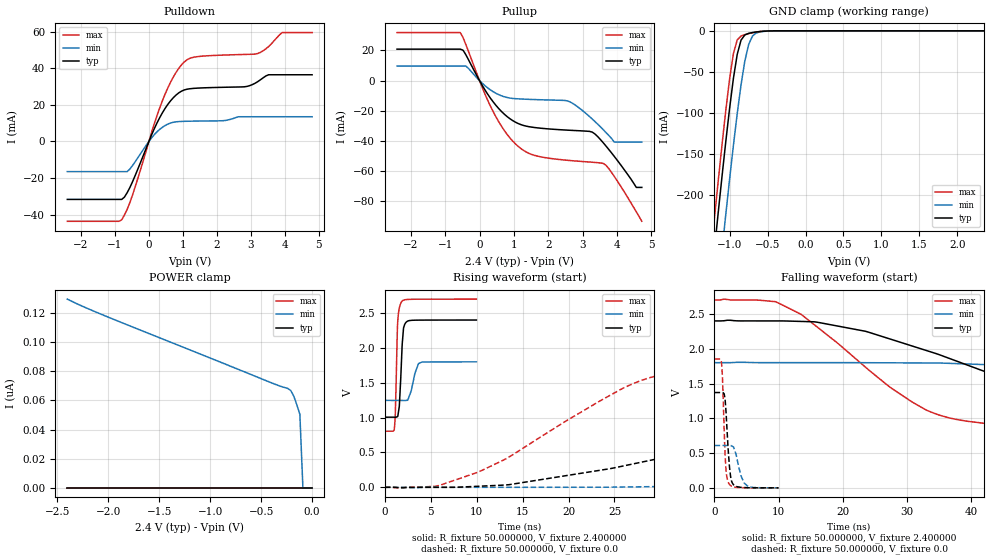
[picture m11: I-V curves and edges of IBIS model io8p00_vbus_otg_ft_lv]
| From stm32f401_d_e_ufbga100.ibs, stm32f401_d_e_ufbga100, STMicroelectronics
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|   Model io8p00_vbus_otg_ft_lv
[Model]  io8p00_vbus_otg_ft_lv
Model_type I/O
Polarity   Non-Inverting
Enable   Active-Low
Vinl =   0.720000V
Vinh =   1.680000V
Vmeas =  1.200000V
Cref =   50.000000pF
Rref =   100.000000M
Vref =   0.0V
C_comp   3.193600pF   3.100000pF   3.332000pF
[Temperature Range]   25.000000   0.125000k   -40.000000
[Pullup Reference]   2.400000V   1.800000V   2.700000V
[Pulldown Reference]   0.0V   0.0V   0.0V
[POWER Clamp Reference]   2.400000V   1.800000V   2.700000V
[GND Clamp Reference]   0.0V   0.0V   0.0V
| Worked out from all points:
|   slope of the pulldown table from 0 to 0.36 V, typ, clamps not added: 25 ohm
|   slope of the pullup table from 0 to 0.36 V, typ, clamps not added: 27.7 ohm
|   GND clamp passes 1 mA (typ) near -0.61 V on its own axis
|   rising waveform, R_fixture 50.000000, V_fixture 2.400000: 20-80 % time 309ps typ, 630ps min, 213ps max; typ from 1.01 V to 2.4 V
|   rising waveform, R_fixture 50.000000, V_fixture 0.0: 20-80 % time 30.9ns typ, 73.2ns min, 14.3ns max; typ from 0 V to 1.37 V
|   falling waveform, R_fixture 50.000000, V_fixture 2.400000: 20-80 % time 29.1ns typ, 72.3ns min, 15.9ns max; typ from 2.4 V to 1.01 V
|   falling waveform, R_fixture 50.000000, V_fixture 0.0: 20-80 % time 575ps typ, 1.04ns min, 436ps max; typ from 1.37 V to 0 V
[Pulldown]
|Voltage   I(typ)   I(min)   I(max)
-2.4V     -31.69mA   -16.5mA    -43.66mA
-800mV    -31.69mA   -16.5mA    -42.82mA
-480mV    -21.96mA   -13.17mA   -29.19mA
80mV      3.63mA     1.966mA    5.014mA
480mV     18.16mA    8.738mA    26.02mA
800mV     25.38mA    10.72mA    37.77mA
1.12V     28.53mA    11.02mA    44.6mA
2.8V      29.84mA    13.49mA    47.53mA
3.2V      32.65mA    13.49mA    48.05mA
3.52V     36.43mA    13.49mA    51.84mA
3.92V     36.43mA    13.49mA    59.49mA
4.8V      36.43mA    13.49mA    59.49mA
[Pullup]
|Voltage   I(typ)   I(min)   I(max)
-2.4V     20.89mA    9.66mA     31.9mA
-560mV    20.89mA    9.66mA     31.9mA
-400mV    17.28mA    9.66mA     24.07mA
320mV     -11.75mA   -6.207mA   -17.08mA
960mV     -26.47mA   -11.82mA   -40.02mA
1.52V     -30.88mA   -12.51mA   -49.05mA
2.56V     -32.88mA   -13.49mA   -52.9mA
3.28V     -34.19mA   -25.52mA   -54.18mA
3.6V      -41.31mA   -32.62mA   -54.99mA
3.92V     -50.33mA   -40.8mA    -63.62mA
4.56V     -70.9mA    -40.8mA    -87.07mA
4.72V     -70.9mA    -40.8mA    -93.4mA
[GND_clamp]
|Voltage   I(typ)   I(min)   I(max)
-2.4V     -1.425A    -1.509A    -1.394A
-1.25V    -311.3mA   -401.9mA   -273.4mA
-1.2V     -265.5mA   -356.1mA   -227.3mA
-1.15V    -220.5mA   -310.9mA   -182mA
-1.1V     -176.4mA   -266.2mA   -138mA
-1.05V    -133.9mA   -222.5mA   -96.06mA
-950mV    -57.51mA   -139mA     -27.35mA
-900mV    -28.55mA   -100.5mA   -11.03mA
-850mV    -11.33mA   -65.67mA   -6.322mA
-750mV    -3.069mA   -16.69mA   -3.425mA
-600mV    -864.6uA   -1.294mA   -852.2uA
2.35V     0A         0A         0A
[POWER_clamp]
|Voltage   I(typ)   I(min)   I(max)
-2.4V     0A         129.4nA    0A
-1.98V    0A         116.5nA    0A
-390mV    0A         71.78nA    0A
-240mV    0A         68.22nA    0A
-210mV    0A         66.81nA    0A
-180mV    0A         62.95nA    0A
-120mV    0A         50.47nA    0A
-90mV     0A         0A         0A
0V        0A         0A         0A
[Ramp]
| variable   typ   min   max
dV/dt_r  0.82302/30.91280n   0.36179/74.96621n   1.11096/14.32018n
dV/dt_f  0.83682/29.15966n   0.32706/74.03173n   1.13770/15.86109n
R_load = 50.000000
[Rising Waveform]
R_fixture= 50.000000
V_fixture= 2.400000
V_fixture_min= 1.800000
V_fixture_max= 2.700000
|time   V(typ)   V(min)   V(max)
0s        1.006V     1.247V     804.6mV
1.041ns   1.006V     1.247V     838mV
1.141ns   1.006V     1.247V     1.039V
1.401ns   1.015V     1.247V     2.359V
1.582ns   1.162V     1.247V     2.571V
1.822ns   1.827V     1.247V     2.66V
2.042ns   2.286V     1.246V     2.685V
2.442ns   2.381V     1.249V     2.695V
3.684ns   2.399V     1.775V     2.699V
9.97ns    2.4V       1.8V       2.7V
[Rising Waveform]
R_fixture= 50.000000
V_fixture= 0.0
V_fixture_min= 0.0
V_fixture_max= 0.0
|time   V(typ)   V(min)   V(max)
0s        6.224nV    371.9nV    2.518nV
5.506ns   -154.1uV   -166.5uV   14.99mV
10.01ns   13.97mV    -63.83uV   210.5mV
28.03ns   363.1mV    7.611mV    1.538V
33.53ns   517.3mV    16.69mV    1.697V
40.54ns   741.8mV    28.24mV    1.777V
60.06ns   1.178V     76.52mV    1.835V
81.08ns   1.32V      193.4mV    1.851V
149.6ns   1.369V     510.6mV    1.852V
249.2ns   1.37V      609.1mV    1.852V
[Falling Waveform]
R_fixture= 50.000000
V_fixture= 2.400000
V_fixture_min= 1.800000
V_fixture_max= 2.700000
|time   V(typ)   V(min)   V(max)
0s        2.4V       1.8V       2.7V
9.51ns    2.4V       1.8V       2.676V
16.02ns   2.381V     1.8V       2.312V
31.03ns   2.033V     1.796V     1.221V
35.54ns   1.897V     1.793V     1.032V
42.54ns   1.66V      1.77V      923.4mV
59.56ns   1.248V     1.713V     845.6mV
87.09ns   1.074V     1.559V     815.4mV
137.6ns   1.017V     1.352V     805.4mV
249.2ns   1.006V     1.247V     804.6mV
[Falling Waveform]
R_fixture= 50.000000
V_fixture= 0.0
V_fixture_min= 0.0
V_fixture_max= 0.0
|time   V(typ)   V(min)   V(max)
0s        1.37V      609.1mV    1.852V
1.061ns   1.37V      609.1mV    1.82V
1.241ns   1.37V      609mV      1.585V
1.682ns   1.237V     608.8mV    423.9mV
2.202ns   464.3mV    608.9mV    68.09mV
2.523ns   157.3mV    609.9mV    32.39mV
3.123ns   32.91mV    547.4mV    12.55mV
4.124ns   7.063mV    174.2mV    3.416mV
5.245ns   1.875mV    19.12mV    498.9uV
9.97ns    6.224nV    371.9nV    2.518nV
